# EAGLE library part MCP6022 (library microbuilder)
MCP6022 - Dual Rail-to-Rail 10MHz Op-Amp Digikey: SOIC8 - MCP6022-I/SN-ND
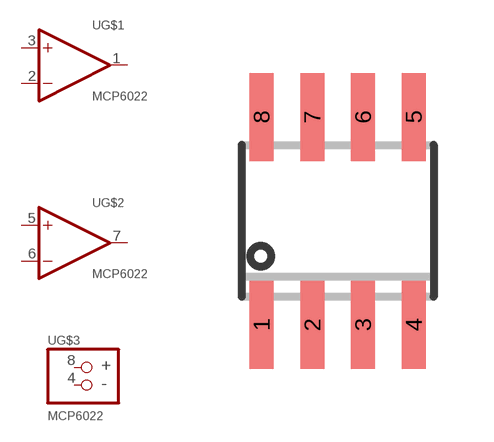
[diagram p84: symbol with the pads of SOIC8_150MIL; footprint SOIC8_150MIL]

Designator prefix U; gates G$1=OPAMP G$2=OPAMP G$3=POWER

## MCP6022  [SOIC8_150MIL]
1  G$1:OUT  out
2  G$1:-IN  in
3  G$1:+IN  in
4  G$3:-  pas
5  G$2:+IN  in
6  G$2:-IN  in
7  G$2:OUT  out
8  G$3:+  pas

## Footprint SOIC8_150MIL (pad centres in mm)
Small Outline IC - 150mil Wide
smd 0.6 x 2.2: 1 -1.905,-2.6; 2 -0.635,-2.6; 3 0.635,-2.6; 4 1.905,-2.6; 5 1.905,2.6; 6 0.635,2.6; 7 -0.635,2.6; 8 -1.905,2.6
